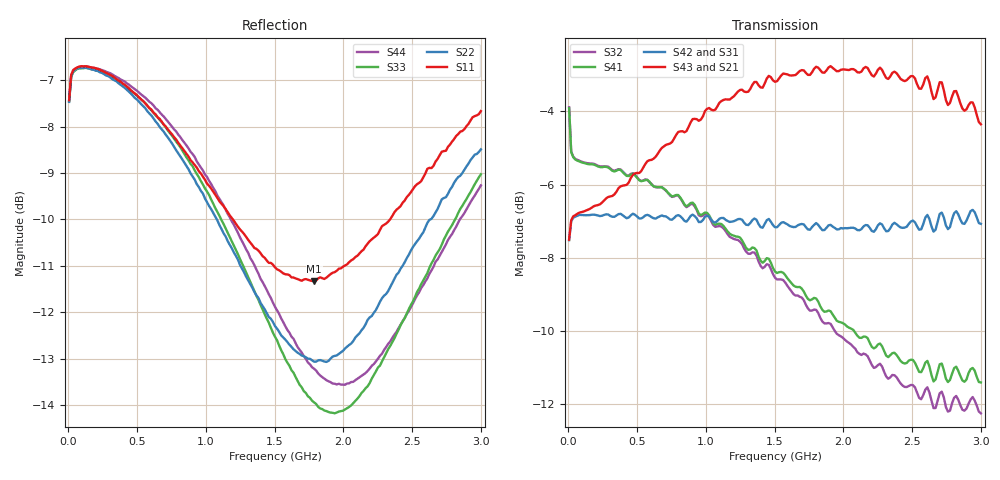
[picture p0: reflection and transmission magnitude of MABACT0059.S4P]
#	MHz	S	RI	R	50
!FREQ	R1	I1	R2	I2	R3	I3	R4	I4
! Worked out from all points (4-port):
!   201 points, 4.5 MHz to 3 GHz, reference 50 ohm
!   strongest paths, dB at 4.5 MHz, 753.4 MHz, 1.502 GHz, 2.251 GHz, 3 GHz:
!     S43: -7.5, -4.8, -3.2, -2.9, -4.4
!     S21: -7.5, -4.8, -3.3, -3.2, -4.7
!     S42: -7.5, -7.0, -7.2, -7.1, -7.1
!     S31: -7.5, -7.1, -7.4, -7.5, -7.4
!     S41: -3.9, -6.3, -8.4, -10.4, -11.4
!     S32: -3.9, -6.3, -8.5, -10.9, -12.2
!   lowest |S11| = -11.3 dB at 1.787 GHz (marker M1), VSWR 1.74, Z = 57 - j29.3 ohm
!   |S11| at or under -10 dB: 1.196 GHz to 2.339 GHz (1.144 GHz wide, 64.7 % of centre)
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4.5  0.3863 0.1773  0.3819 0.18  -0.3865 -0.169  0.6113 -0.1761
     0.3804 0.1804  0.3833 0.1796  0.6131 -0.1762  -0.3877 -0.1668
     -0.3849 -0.1693  0.6144 -0.1768  0.3877 0.1716  0.3879 0.1689
     0.6129 -0.1761  -0.3862 -0.1674  0.3861 0.1695  0.3882 0.173
34.455  0.4578 0.0173  0.4527 0.0363  -0.4508 -0.0102  0.5432 -0.0551
        0.4529 0.0364  0.4563 0.0152  0.5443 -0.0531  -0.4511 -0.00912
        -0.451 -0.0102  0.545 -0.053  0.4555 0.0147  0.4518 0.035
        0.5435 -0.0555  -0.4515 -0.00919  0.4523 0.035  0.4567 0.0154
154.275  0.4569 -0.0651  0.4648 0.0261  -0.4465 0.0865  0.5236 -0.1067
         0.4646 0.0267  0.4538 -0.0732  0.5268 -0.0982  -0.4469 0.0895
         -0.4466 0.0861  0.5269 -0.0976  0.454 -0.0712  0.4637 0.0242
         0.5237 -0.1059  -0.4466 0.0894  0.4636 0.0248  0.4562 -0.0694
798.3075  0.2769 -0.2639  0.588 0.000427  -0.2276 0.386  0.2856 -0.3892
          0.5905 0.00061  0.2425 -0.283  0.3152 -0.3645  -0.2157 0.3987
          -0.2295 0.387  0.317 -0.366  0.2464 -0.2906  0.5892 -0.00647
          0.2876 -0.3907  -0.2166 0.4006  0.5916 -0.00616  0.2576 -0.2933
1786.822  0.1307 -0.2375  0.6335 -0.3163  0.2144 0.3715  -0.1545 -0.317
          0.632 -0.3091  0.0832 -0.206  -0.0995 -0.3248  0.2535 0.363
          0.2106 0.3699  -0.0978 -0.3238  0.0547 -0.1932  0.635 -0.3491
          -0.1518 -0.3165  0.2513 0.3632  0.6349 -0.3434  0.0455 -0.2135
2610.585  0.1156 -0.3394  0.4024 -0.5329  0.4102 0.142  -0.2803 -0.0522
          0.4222 -0.5312  0.0935 -0.2992  -0.248 -0.0823  0.4397 0.0961
          0.4113 0.1536  -0.2498 -0.0883  0.0838 -0.2637  0.3695 -0.5879
          -0.2819 -0.0584  0.4435 0.1046  0.3822 -0.5919  0.0527 -0.268
3000  0.0411 -0.4117  0.2611 -0.5132  0.4247 0.0142  -0.2586 0.0683
      0.2735 -0.5131  0.0209 -0.3757  -0.239 0.0431  0.4393 -0.0438
      0.4271 0.022  -0.2408 0.0402  0.0175 -0.3533  0.2039 -0.5677
      -0.2616 0.0627  0.4416 -0.0367  0.2145 -0.5668  -0.0191 -0.3435
